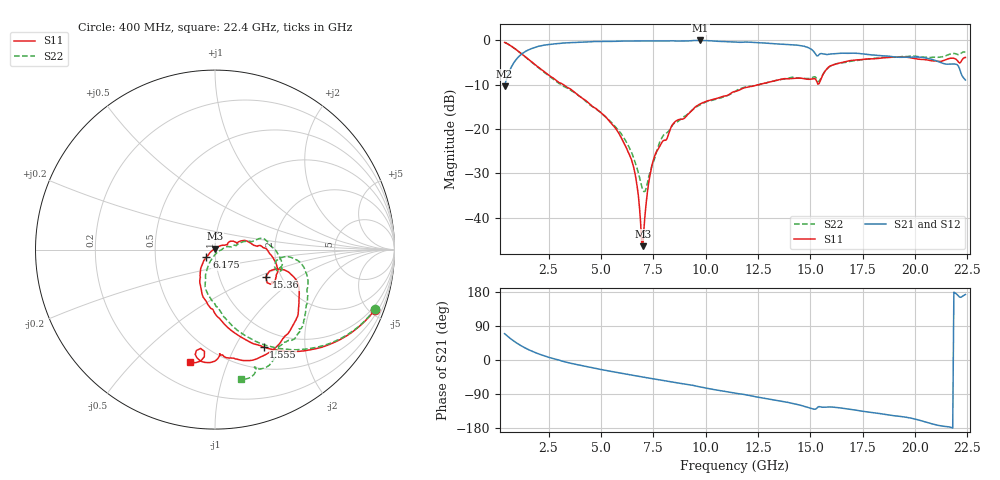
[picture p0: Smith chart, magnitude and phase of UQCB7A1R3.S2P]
!  Part Number  UQCB7A1R3  Mounting Orientation: Vertical
!  Description: RF capacitors
!  Application: Coupling, Bypass, Tuning, DC Block
!  Filters, Matching
# GHZ S DB R 50
! Freq  |S11|  S11 Ph  |S21|  S21 Ph  |S12|  S12 Ph  |S22|  S22 Ph
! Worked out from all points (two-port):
!   401 points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, 400 MHz to 22.4 GHz, reference 50 ohm
!   highest |S21| = 0.00 dB at 9.75 GHz (marker M1); lowest = -10.3 dB at 400 MHz (marker M2)
!   |S21| within 3 dB of the highest: 1.234 GHz to 15.24 GHz (14 GHz wide, 170 % of centre); 16.07 GHz to 17.43 GHz (1.357 GHz wide, 8.1 % of centre)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
!   lowest |S11| = -46.4 dB at 7 GHz (marker M3), VSWR 1.01, Z = 49.9 + j0.476 ohm
!   |S11| at or under -10 dB: 3.212 GHz to 12.5 GHz (9.288 GHz wide, 118 % of centre)
!   |S22| runs from -34.1 to -0.4 dB; largest |S21 - S12| = 0.0051
!   S11 on the Smith chart (normalised r, x): 400 MHz: 0.77, -5.38; 1.555 GHz: 0.76, -1.31; 6.175 GHz: 0.91, -0.08; 15.36 GHz: 1.67, -0.56; 22.4 GHz: 0.35, -0.74
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0.4  -0.44 -20.6  -10.32 69.4  -10.35 69.4  -0.43 -20.2
0.895  -1.86 -42.3  -4.66 47.8  -4.67 47.9  -1.86 -41.5
1.555  -4.34 -63.5  -2.09 26.9  -2.11 26.9  -4.35 -61.8
2.49  -7.76 -83.7  -0.92 7.3  -0.94 7.3  -7.91 -80.1
4.085  -12.95 -110.4  -0.39 -14.8  -0.40 -14.7  -12.97 -103.1
6.175  -23.87 -138.1  -0.14 -36.9  -0.13 -36.8  -22.60 -111.9
6.615  -29.79 -149.0  -0.11 -41.3  -0.10 -41.1  -27.25 -104.9
6.89  -40.87 -179.1  -0.11 -43.9  -0.11 -43.8  -31.85 -85.2
7  -46.40 96.0  -0.11 -45.0  -0.10 -44.8  -33.82 -66.7
7.385  -29.36 36.7  -0.11 -48.6  -0.10 -48.5  -29.11 -1.7
7.77  -24.15 24.3  -0.11 -52.3  -0.09 -52.1  -23.39 13.9
8.485  -18.60 22.0  -0.10 -59.1  -0.08 -58.9  -18.72 11.7
9.75  -14.27 12.6  0.00 -71.3  -0.01 -71.1  -14.48 14.1
11.4  -11.51 2.8  -0.34 -87.6  -0.33 -87.5  -11.50 13.7
14.04  -8.62 -23.0  -0.95 -113.2  -0.94 -113.2  -8.39 -10.9
15.085  -8.68 -29.4  -2.14 -128.6  -2.13 -128.7  -8.37 -15.1
15.36  -9.87 -28.2  -3.47 -124.2  -3.46 -124.1  -9.23 -16.2
16.075  -5.51 -27.6  -3.00 -124.4  -3.01 -124.5  -5.53 -15.1
18.77  -3.81 -59.9  -3.56 -145.2  -3.54 -145.4  -3.74 -42.1
20.75  -4.57 -85.7  -4.20 -167.5  -4.20 -167.7  -3.83 -54.2
21.905  -4.12 -97.9  -5.33 177.3  -5.31 177.1  -2.96 -69.3
22.4  -3.84 -102.8  -8.92 172.9  -8.91 172.6  -2.67 -78.8
